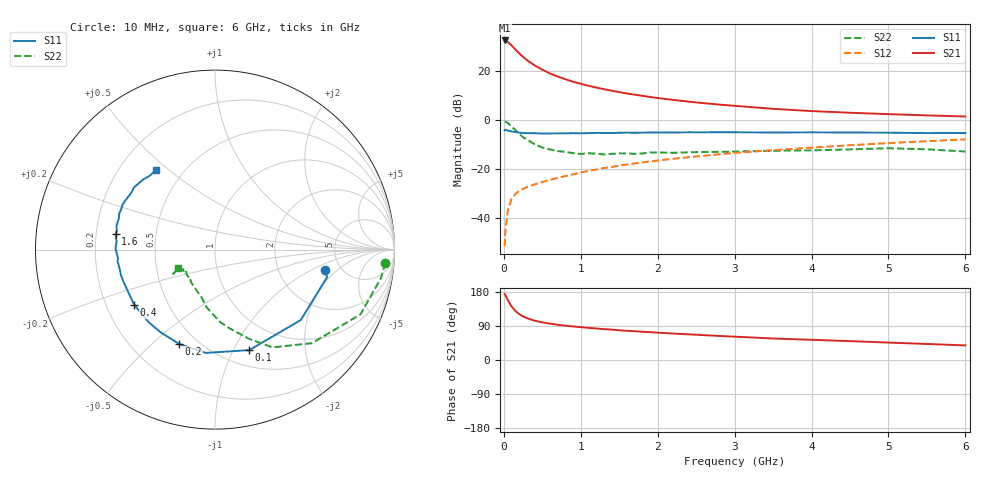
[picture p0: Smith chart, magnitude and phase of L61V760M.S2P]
!  INFINEON TECHNOLOGIES Small Signal Semiconductors
! BFR380L3 , Si-NPN RF-Transistor in TSLP-3-1
!  Vce=1.75 V,  Ic=60 mA
! Common Emitter S-Parameters:  07. March 2005
#  GHz  S  MA  R  50
! f  S11  S21  S12  S22
! GHz  Mag  Ang  Mag  Ang  Mag  Ang  Mag  Ang
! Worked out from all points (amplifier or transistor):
!   36 points, 10 MHz to 6 GHz, reference 50 ohm
!   highest |S21| = 32.6 dB at 10 MHz (marker M1)
!   |S21| within 3 dB of that: start of sweep to 129.4 MHz
!   unconditionally stable (mu >= 1): 1.338 GHz to 4.943 GHz
!   at 250 MHz: K = 0.50, MSG = 26.9 dB, |S12| = -28.0 dB
!   at 1.4 GHz: K = 1.01, MAG = 15.0 dB, |S12| = -19.0 dB
!   at 6 GHz: K = 0.98, MSG = 4.7 dB, |S12| = -7.8 dB
!   S11 on the Smith chart (normalised r, x): 10 MHz: 3.74, -1.42; 100 MHz: 0.67, -1.16; 200 MHz: 0.40, -0.61; 400 MHz: 0.32, -0.28; 1.6 GHz: 0.28, +0.07; 6 GHz: 0.35, +0.45
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0.01  0.6235 -10.7  42.68 173.9  0.0027 78.1  0.952 -4.5
0.02  0.6432 -13.8  42.36 171.5  0.0053 86.3  0.9379 -9.8
0.05  0.6184 -39.4  39.93 158.6  0.014 73.7  0.8872 -24.0
0.1  0.5915 -71.2  33.8 141.5  0.0251 61.8  0.7506 -44.0
0.15  0.578 -95.2  27.94 129.3  0.0314 56.1  0.6323 -59.5
0.2  0.5618 -111.1  23.25 121.0  0.0365 53.9  0.5321 -69.1
0.25  0.5515 -123.3  19.75 115.0  0.04 51.4  0.4505 -78.9
0.3  0.548 -132.3  16.96 110.4  0.0434 51.8  0.4049 -85.9
0.4  0.5451 -145.7  13.24 103.7  0.0492 52.5  0.3253 -98.2
0.5  0.5382 -154.0  10.8 99.4  0.0552 54.4  0.278 -105.4
0.6  0.54 -160.3  9.046 95.8  0.0605 56.7  0.2542 -112.6
0.7  0.543 -164.6  7.837 93.1  0.067 58.3  0.2359 -119.6
0.9  0.5465 -173.1  6.135 88.5  0.0792 61.5  0.2142 -130.2
1.1  0.5485 -178.1  5.076 84.8  0.0929 63.4  0.213 -135.0
1.3  0.552 176.8  4.331 81.4  0.1062 64.1  0.2013 -142.4
1.6  0.5611 170.9  3.537 77.1  0.1257 64.9  0.2114 -148.0
2.2  0.5631 162.1  2.615 69.8  0.1644 65.5  0.2175 -149.2
2.8  0.5728 154.0  2.098 63.5  0.2027 65.3  0.2272 -153.8
3.5  0.5638 145.8  1.717 56.7  0.2456 63.0  0.2398 -152.0
4.5  0.5641 139.6  1.428 49.8  0.31 61.0  0.2551 -150.8
5.5  0.5489 131.4  1.26 42.3  0.375 56.8  0.2561 -150.8
6  0.5522 126.5  1.197 38.5  0.4078 54.6  0.2306 -154.1
